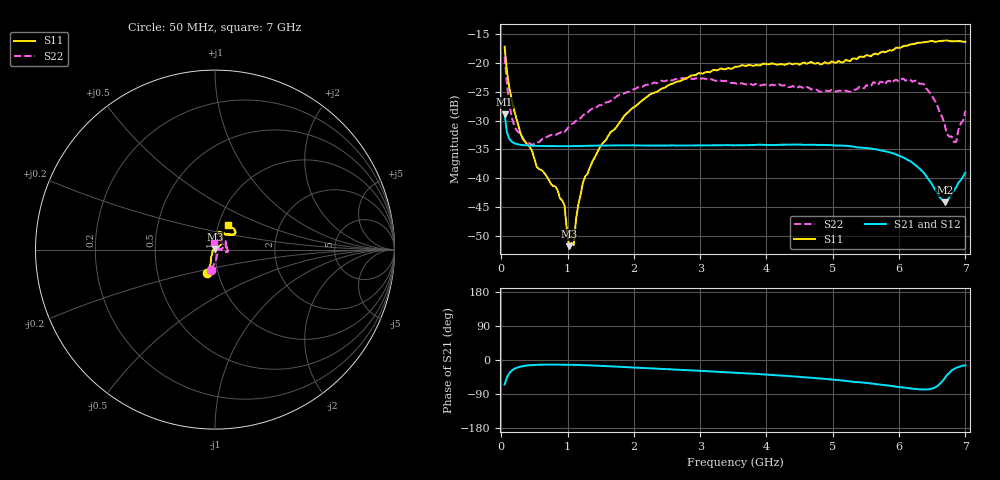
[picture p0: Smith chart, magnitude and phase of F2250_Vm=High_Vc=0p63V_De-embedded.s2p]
! Integrated Device Technology
! Corporate Headquarters
! 6024 Silver Creek Valley Road
! San Jose, CA 95138  USA
! Phone:  1-408-284-8200
! Toll Free:  1-800-223-1366
! Webpage:  http://www.idt.com/
! Timing and RF Division
! 515 Groton Road, Suite 102
! Westford, MA 01886-6024
! Device:  F2250
! Description: Voltage Variable RF Attenuator
! Frequency:  50.0 -  6000.00 MHz
! Package:  3x3 mm Thin QFN Plastic Package: 16 pin
! Ports:  2 RF, 3 DC
!  Pin  1  = GND
!  Pin  2  = NC
!  Pin  3  = RF1  = Port 1
!  Pin  4  = NC
!  Pin  5  = GND
!  Pin  6  = GND
!  Pin  7  = GND
!  Pin  8  = GND
!  Pin  9  = NC
!  Pin 10  = RF2  = Port 2
!  Pin 11  = NC
!  Pin 12  = GND
!  Pin 13  = GND
!  Pin 14  = VCNTRL
!  Pin 15  = VDD
!  Pin 16  = VMODE
! Vcntrl:  0.630 Volts
! Vmode:  +3.300 Volts
! Vdd:  +3.30  Volts
! Current:  1.279 mA
! Data:  The device was measured on a the F2250 evaluation board which has
!  individual transmission lines to the RF pins.  Data was collected
!  using a calibrated network analyzer.  The evaluation board was
!  de-embedded using a TRL calibration technique.
!  The reference plane is the edge of the package pin.
! Misc:  SN 10
!  Action Tracker AT0258
! Date Measured:  2014-11-26
! Date:  2015-10-15  MJV
! Note:
!  Integrated Device Technology supplies this data as a sample of measured
!  data at the package pin for this product.  Your particular data for this
!  product may vary.
!  Data was taken at 25 degrees C.
!  Integrated Device Technology reserves the right to change this data at anytime.
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# GHz S dB R 50
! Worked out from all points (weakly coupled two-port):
!   201 points, 50 MHz to 7 GHz, reference 50 ohm
!   highest |S21| = -28.90 dB at 50 MHz (marker M1); lowest = -44.2 dB at 6.687 GHz (marker M2)
!   lowest |S11| = -51.8 dB at 1.023 GHz (marker M3), VSWR 1.01, Z = 49.8 + j0.171 ohm
!   |S11| at or under -10 dB: start of sweep to end of sweep
!   |S22| runs from -34.2 to -18.9 dB; largest |S21 - S12| = 6.1e-05
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0.05  -17.17 -108.3  -28.90 -64.8  -28.91 -64.7  -18.93 -101.3
0.08475  -21.46 -107.1  -32.02 -46.0  -32.02 -46.0  -23.66 -86.2
0.15425  -26.23 -116.2  -33.62 -28.5  -33.62 -28.4  -29.24 -72.0
0.29325  -32.32 -126.7  -34.20 -17.3  -34.20 -17.3  -32.33 -42.6
0.36275  -33.69 -138.9  -34.28 -15.1  -34.28 -15.1  -33.63 -26.7
0.5365  -38.05 -153.8  -34.38 -12.7  -34.37 -12.7  -33.73 -10.6
0.8145  -41.40 170.3  -34.42 -12.1  -34.42 -12.1  -32.52 1.5
0.9535  -44.70 171.4  -34.43 -12.4  -34.43 -12.4  -31.95 4.2
1.023  -51.76 138.2  -34.42 -12.6  -34.42 -12.6  -30.96 5.9
1.0925  -51.59 83.3  -34.41 -12.9  -34.41 -12.9  -30.44 7.6
1.12725  -47.10 57.7  -34.40 -13.0  -34.40 -13.0  -30.01 6.6
1.2315  -40.71 38.9  -34.37 -13.5  -34.37 -13.5  -29.11 5.9
1.6485  -31.98 40.5  -34.31 -16.7  -34.32 -16.7  -26.59 14.6
2.37825  -24.75 46.3  -34.31 -23.1  -34.31 -23.1  -23.34 24.9
3.525  -20.67 71.5  -34.28 -33.6  -34.29 -33.6  -23.50 53.2
4.7065  -20.08 71.9  -34.19 -47.4  -34.19 -47.4  -24.58 57.4
5.2625  -19.68 53.1  -34.43 -56.4  -34.43 -56.5  -25.02 33.4
5.85325  -17.80 40.5  -35.50 -67.9  -35.51 -68.0  -23.08 5.0
6.3745  -16.41 40.9  -39.07 -78.0  -39.08 -78.0  -23.68 -11.8
6.68725  -16.13 47.8  -44.16 -48.2  -44.16 -47.9  -30.68 7.3
6.861  -16.23 54.4  -41.55 -20.8  -41.51 -20.8  -33.70 62.0
7  -16.34 62.4  -39.02 -14.0  -39.00 -14.1  -28.29 101.4
